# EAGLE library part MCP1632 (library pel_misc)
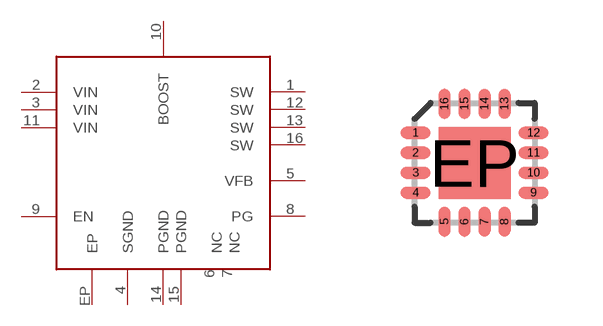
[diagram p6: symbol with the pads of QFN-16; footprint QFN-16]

Designator prefix IC

## MCP1632  [QFN-16]
1  SW
2  VIN
3  VIN
4  SGND
5  VFB
6  NC
7  NC
8  PG
9  EN
10  BOOST
11  VIN
12  SW
13  SW
14  PGND
15  PGND
16  SW
EP  EP

## Footprint QFN-16 (pad centres in mm)
smd 0.75 x 0.3: 1 -1.475,0.75; 2 -1.475,0.25; 3 -1.475,-0.25; 4 -1.475,-0.75; 9 1.475,-0.75; 10 1.475,-0.25; 11 1.475,0.25; 12 1.475,0.75
smd 0.3 x 0.75: 5 -0.75,-1.475; 6 -0.25,-1.475; 7 0.25,-1.475; 8 0.75,-1.475; 13 0.75,1.475; 14 0.25,1.475; 15 -0.25,1.475; 16 -0.75,1.475
smd 1.8 x 1.8: EP 0,0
